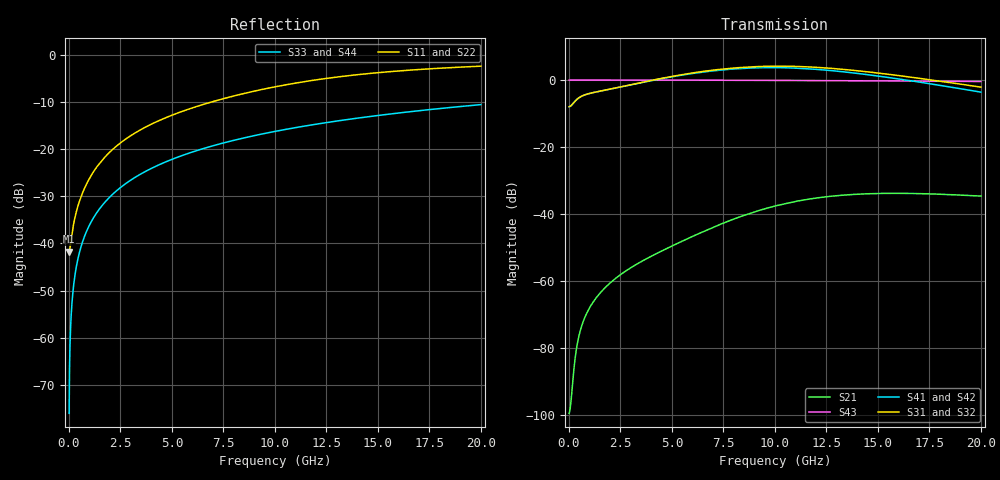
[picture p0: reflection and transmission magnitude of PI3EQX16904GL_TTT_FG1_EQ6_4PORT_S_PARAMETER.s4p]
! NPort=4 DATA=2000 NOISE=0 GROUPDELAY=0 COMPLEX_DATAFORMAT=POLAR
! NumOfBlock=1 NumOfParam=0
! .MODEL Smodel S TSTONEFILE=PI3EQX16904GL_TTT_FG1_EQ6_4PORT_S_PARAMETER.s4p TYPE=S
!  -- The above .MODEL line can be used for the S element in the netlist.
! The s parameter is extracted from the linear redriver, it is not bi-directional; only s(4,1)s(4,2) and s(3,1)s(3,2)
! should be the insertion loss
!Port definition:
!Port1 = input+
!Port2 = input-
!Port3 = output+
!Port4 = output-
# Hz S MA R  50
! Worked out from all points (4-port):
!   2000 points, 10 MHz to 20 GHz, reference 50 ohm
!   strongest paths, dB at 10 MHz, 5.01 GHz, 10.01 GHz, 15.01 GHz, 20 GHz:
!     S31: -8.0, 1.1, 4.1, 2.1, -2.1
!     S32: -8.0, 1.0, 4.0, 1.9, -2.3
!     S41: -8.0, 1.0, 3.7, 1.2, -3.6
!     S42: -8.0, 0.9, 3.6, 1.0, -3.8
!     S43: 0.0, 0.0, -0.1, -0.3, -0.4
!     S21: -99.6, -49.6, -37.6, -33.9, -34.7
!   lowest |S11| = -41.7 dB at 10 MHz (marker M1), VSWR 1.02, Z = 49.2 - j0.0603 ohm
!   |S11| at or under -10 dB: start of sweep to 6.871 GHz
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1e7  0.008182 -175.7  1.05e-05 7.8  0 0.0  0 0.0
     1.05e-05 7.8  0.008182 -175.7  0 0.0  0 0.0
     0.3996 0.7  0.3996 -179.3  0.0001571 -90.0  1 -0.0
     0.3996 -179.3  0.3996 0.7  1 -0.0  0.0001571 -90.0
3.8e8  0.02256 -119.7  0.0001024 118.3  0 0.0  0 0.0
       0.0001024 118.3  0.02256 -119.7  0 0.0  0 0.0
       0.5117 13.7  0.5117 -166.4  0.005969 -90.4  1 -0.3
       0.5117 -167.0  0.5116 12.9  1 -0.3  0.005969 -90.4
1.6e9  0.07608 -102.8  0.0007037 109.1  0 0.0  0 0.0
       0.0007034 109.1  0.07608 -102.8  0 0.0  0 0.0
       0.6909 5.4  0.6912 -174.8  0.02512 -91.5  0.9997 -1.4
       0.69 -177.4  0.6903 2.3  0.9997 -1.4  0.02512 -91.5
5.88e9  0.2705 -104.6  0.004468 101.3  0 0.0  0 0.0
        0.004434 101.6  0.2705 -104.6  0 0.0  0 0.0
        1.259 -36.7  1.244 142.5  0.09194 -95.5  0.9954 -5.3
        1.237 132.8  1.222 -47.9  0.9954 -5.3  0.09194 -95.5
9.65e9  0.4449 -111.9  0.01236 70.5  0 0.0  0 0.0
        0.01226 71.4  0.4447 -111.9  0 0.0  0 0.0
        1.604 -97.0  1.579 82.4  0.1497 -99.0  0.9878 -8.6
        1.532 66.2  1.509 -114.4  0.9878 -8.6  0.1497 -99.0
1.372e10  0.6112 -122.5  0.01954 21.1  0 0.0  0 0.0
          0.01944 22.5  0.6109 -122.4  0 0.0  0 0.0
          1.404 -164.2  1.38 15.2  0.2103 -102.6  0.9758 -12.1
          1.285 -7.4  1.263 172.0  0.9758 -12.1  0.2103 -102.6
2e10  0.7646 -136.3  0.01845 -36.7  0 0.0  0 0.0
      0.01845 -34.7  0.7648 -136.3  0 0.0  0 0.0
      0.783 111.2  0.7664 -69.4  0.2986 -108.1  0.9506 -17.4
      0.6593 -100.8  0.6453 78.7  0.9506 -17.4  0.2986 -108.1
